PROGRAM PRG_Slow
VAR
		fbTxtParser	: FB_TxtParser;
END_VAR



fbTxtParser(bExecute:= , 
	sFilePathSource:= , 
	sFilePathDestination:= , 
	eMode:= , 
	nParsePerCycle:= nAcquisitionBlock, 
	bBusy=> , 
	bError=> , 
	nErrId=> );

fbTxtParser.bExecute := false;

END_PROGRAM
